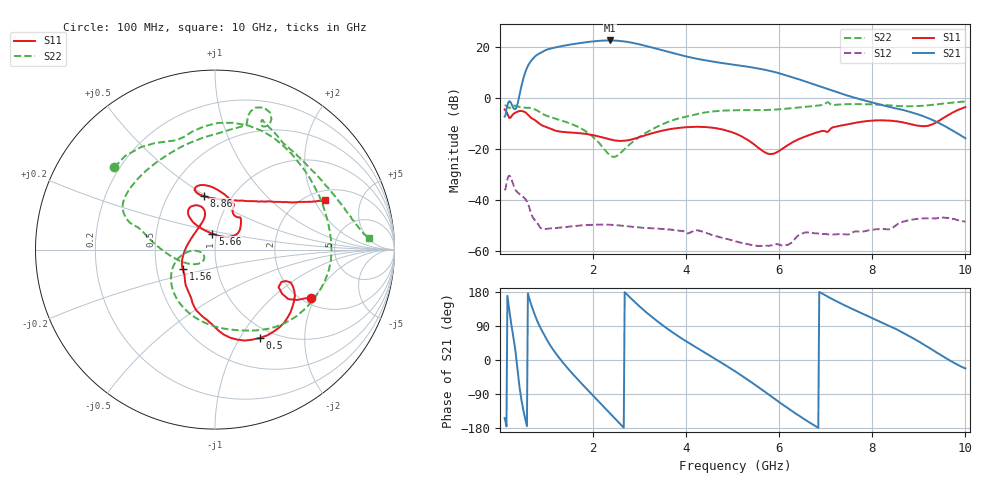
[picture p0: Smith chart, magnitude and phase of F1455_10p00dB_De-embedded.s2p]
! Integrated Device Technology
! Corporate Headquarters
! 6024 Silver Creek Valley Road
! San Jose, CA 95138  USA
! Phone:  1-408-284-8200
! Toll Free:  1-800-223-1366
! Webpage:  http://www.idt.com/
! Timing and RF Division
! 515 Groton Road, Suite 102
! Westford, MA 01886-6024
! Device:  F1455
! Description: 6-bit 0.5 dB Transmit Variable Gain Amplifier
! Frequency:  1400.0 -  2300.00 MHz
! Package:  6x6 mm Thin QFN Plastic Package: 28 pin
! State:  20
! Atten State:  10.0 dB
! Voltage:  +5.00 Volts
! Current:  217.678 mA
! Data:  The device was measured on a the F1455 evaluation board which has
!  individual transmission lines to the RF pins.  Data was collected
!  using a calibrated network analyzer.  The evaluation board was
!  de-embedded using a TRL calibration technique.
!  The reference plane is the edge of the package pin.
!  Pin  1 = CSb
!  Pin  2 = DATA
!  Pin  3 = CLK
!  Pin  4 = RSET
!  Pin  5 = GND
!  Pin  6 = RFIN  = Port 1
!  Pin  7 = GND
!  Pin  8 = NC
!  Pin  9 = NC
!  Pin 10 = NC
!  Pin 11 = NC
!  Pin 12 = NC
!  Pin 13 = NC
!  Pin 14 = /STBY
!  Pin 15 = GND
!  Pin 16 = RFOUT  = Port 2
!  Pin 17 = GND
!  Pin 18 = NC
!  Pin 19 = NC
!  Pin 20 = NC
!  Pin 21 = GND
!  Pin 22 = NC
!  Pin 23 = GND
!  Pin 24 = NC
!  Pin 25 = NC
!  Pin 26 = NC
!  Pin 27 = GND
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# GHz S dB R 50
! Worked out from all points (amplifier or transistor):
!   496 points, 100 MHz to 10 GHz, reference 50 ohm
!   highest |S21| = 22.7 dB at 2.36 GHz (marker M1)
!   |S21| within 3 dB of that: 1.13 GHz to 3.313 GHz (2.183 GHz wide, 98.2 % of centre)
!   unconditionally stable (mu >= 1): start of sweep to end of sweep
!   at 1.74 GHz: K = 11.59, MAG = 22.3 dB, |S12| = -50.0 dB
!   at 5.06 GHz: K = 45.96, MAG = 15.1 dB, |S12| = -56.3 dB
!   at 10 GHz: K = 115.84, MAG = -7.2 dB, |S12| = -48.6 dB
!   S11 on the Smith chart (normalised r, x): 100 MHz: 2.23, -1.88; 500 MHz: 0.86, -1.22; 1.56 GHz: 0.68, -0.16; 5.66 GHz: 0.96, +0.17; 8.86 GHz: 0.74, +0.49; 10 GHz: 2.42, +2.43
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0.1  -4.42 -26.6  -7.20 -153.3  -36.21 44.5  -2.80 140.8
0.38  -5.25 -39.5  -2.14 -29.7  -37.09 -112.4  -3.20 56.6
0.5  -5.17 -63.2  7.62 -130.7  -38.83 -150.3  -3.70 27.5
0.68  -7.81 -94.1  14.96 142.8  -45.85 148.4  -3.91 -15.2
0.8  -9.27 -109.1  17.12 103.5  -48.99 133.5  -4.82 -43.5
0.94  -10.95 -120.6  18.57 68.7  -51.51 124.5  -6.37 -69.8
1.24  -12.92 -138.4  20.19 10.7  -50.98 90.5  -8.31 -110.8
1.56  -13.56 -148.6  21.28 -36.4  -50.39 59.8  -10.30 -142.9
1.76  -13.83 -155.1  21.83 -63.0  -50.01 44.2  -12.05 -158.3
2.06  -14.75 -168.1  22.48 -101.6  -49.72 23.8  -16.25 -175.0
2.36  -16.16 169.9  22.75 -140.3  -49.79 5.2  -22.39 -165.7
2.54  -16.77 152.1  22.61 -163.3  -50.02 -4.7  -22.31 -141.1
2.74  -16.54 131.8  22.17 171.7  -50.38 -14.4  -18.90 -138.2
3.06  -14.96 110.5  20.94 134.7  -50.93 -27.0  -14.47 -158.0
3.4  -13.13 105.1  19.32 100.5  -51.35 -38.7  -11.01 -177.7
4.08  -11.34 115.1  16.11 43.3  -52.93 -58.3  -6.94 163.7
5.06  -13.87 128.8  13.11 -30.5  -56.35 -96.6  -4.70 148.2
5.66  -20.95 99.7  11.32 -81.1  -58.20 -98.8  -4.65 124.0
6.7  -14.13 43.3  5.75 -168.7  -52.92 -137.0  -3.12 78.3
8.36  -8.78 107.2  -3.39 89.9  -51.56 164.7  -2.78 62.1
8.86  -10.29 101.8  -5.63 58.4  -47.79 147.3  -3.15 42.6
10  -3.47 24.3  -15.75 -22.2  -48.59 73.9  -1.29 4.4
